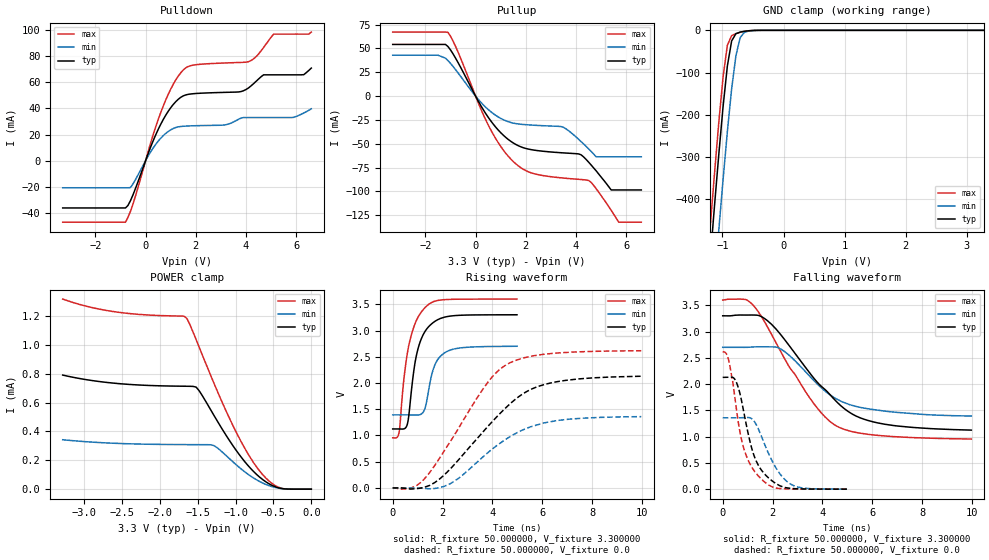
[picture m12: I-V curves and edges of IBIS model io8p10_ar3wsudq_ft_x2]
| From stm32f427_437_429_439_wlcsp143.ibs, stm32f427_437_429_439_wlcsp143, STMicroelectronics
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|   Model io8p10_ar3wsudq_ft_x2
[Model]  io8p10_ar3wsudq_ft_x2
Model_type I/O
Polarity   Non-Inverting
Enable   Active-Low
Vinl =   0.990000V
Vinh =   2.310000V
Vmeas =  1.650000V
Cref =   40.000000pF
Rref =   100.000000M
Vref =   0.0V
C_comp   7.528700pF   7.342900pF   7.752900pF
[Temperature Range]   25.000000   0.125000k   -40.000000
[Pullup Reference]   3.300000V   2.700000V   3.600000V
[Pulldown Reference]   0.0V   0.0V   0.0V
[POWER Clamp Reference]   3.300000V   2.700000V   3.600000V
[GND Clamp Reference]   0.0V   0.0V   0.0V
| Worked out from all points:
|   slope of the pulldown table from 0 to 0.495 V, typ, clamps not added: 20.9 ohm
|   slope of the pullup table from 0 to 0.495 V, typ, clamps not added: 22.6 ohm
|   GND clamp passes 1 mA (typ) near -0.57 V on its own axis
|   rising waveform, R_fixture 50.000000, V_fixture 3.300000: 20-80 % time 482ps typ, 432ps min, 512ps max; typ from 1.12 V to 3.3 V
|   rising waveform, R_fixture 50.000000, V_fixture 0.0: 20-80 % time 2.52ns typ, 2.27ns min, 2.13ns max; typ from 0 V to 2.13 V
|   falling waveform, R_fixture 50.000000, V_fixture 3.300000: 20-80 % time 2.35ns typ, 1.93ns min, 2.08ns max; typ from 3.3 V to 1.12 V
|   falling waveform, R_fixture 50.000000, V_fixture 0.0: 20-80 % time 718ps typ, 844ps min, 663ps max; typ from 2.13 V to 0 V
[Pulldown]
|Voltage   I(typ)   I(min)   I(max)
-3.3V     -36.18mA   -20.77mA   -47.07mA
-800mV    -36.18mA   -20.77mA   -47.07mA
-600mV    -30.5mA    -20.52mA   -38.69mA
700mV     31.4mA     19.11mA    41.71mA
1.2V      45.15mA    25.37mA    61.75mA
1.6V      50.35mA    26.5mA     71.06mA
3.1V      52.28mA    27.26mA    74.75mA
4.1V      55.71mA    33.01mA    75.8mA
4.7V      65.73mA    33.01mA    86.69mA
5.1V      65.73mA    33.01mA    96.9mA
6.3V      65.85mA    36.5mA     96.9mA
6.6V      70.91mA    39.71mA    98.45mA
[Pullup]
|Voltage   I(typ)   I(min)   I(max)
-3.3V     54.22mA    42.91mA    67.16mA
-1.1V     51.99mA    37.3mA     66.87mA
500mV     -22.07mA   -14mA      -30.03mA
1.5V      -49.1mA    -28.3mA    -68.56mA
2.2V      -56.05mA   -30.32mA   -80.35mA
3.5V      -59.53mA   -32.72mA   -85.92mA
4.2V      -61.52mA   -47.7mA    -87.46mA
4.5V      -69.21mA   -55.3mA    -88.43mA
4.8V      -78.3mA    -63.6mA    -97.02mA
5.4V      -98.4mA    -63.6mA    -119.8mA
5.7V      -98.4mA    -63.6mA    -132.2mA
6.6V      -98.4mA    -63.6mA    -132.2mA
[GND_clamp]
|Voltage   I(typ)   I(min)   I(max)
-3.3V     -4.652A    -4.81A     -4.601A
-1.2V     -540.3mA   -722.7mA   -464.2mA
-1.13V    -414.5mA   -596.2mA   -338mA
-1.06V    -293.4mA   -472.4mA   -217.6mA
-990mV    -180.4mA   -352.9mA   -109.9mA
-920mV    -84.42mA   -240mA     -35.36mA
-850mV    -25.15mA   -138.9mA   -12.53mA
-780mV    -7.942mA   -60.01mA   -7.772mA
-710mV    -4.199mA   -17.23mA   -4.763mA
-640mV    -2.296mA   -4.566mA   -2.439mA
-570mV    -1.048mA   -1.643mA   -953.6uA
3.28V     0A         0A         0A
[POWER_clamp]
|Voltage   I(typ)   I(min)   I(max)
-3.28V    790.5uA    342.5uA    1.317mA
-2.6V     734.3uA    318.1uA    1.23mA
-1.68V    713.4uA    308.8uA    1.199mA
-1.64V    713.1uA    308.7uA    1.182mA
-1.52V    707.2uA    308.5uA    1.037mA
-1.48V    682.1uA    308.4uA    984.7uA
-1.28V    507.2uA    300.7uA    728.4uA
-960mV    246.2uA    155.1uA    363.1uA
-720mV    101uA      64.07uA    152.4uA
-560mV    37.87uA    24.53uA    57.3uA
-440mV    10.21uA    7.381uA    14.65uA
0V        0A         0A         0A
[Ramp]
| variable   typ   min   max
dV/dt_r  1.26570/2.50561n   0.80886/2.25031n   1.56324/2.12207n
dV/dt_f  1.28142/2.33437n   0.77238/1.90340n   1.57424/2.07286n
R_load = 50.000000
[Rising Waveform]
R_fixture= 50.000000
V_fixture= 3.300000
V_fixture_min= 2.700000
V_fixture_max= 3.600000
|time   V(typ)   V(min)   V(max)
0s        1.124V     1.392V     954.2mV
260.3ps   1.124V     1.392V     1.069V
430.4ps   1.124V     1.392V     1.99V
570.6ps   1.19V      1.392V     2.517V
720.7ps   1.722V     1.391V     2.868V
940.9ps   2.503V     1.389V     3.182V
1.301ns   2.986V     1.528V     3.439V
1.672ns   3.168V     2.323V     3.555V
2.082ns   3.255V     2.575V     3.588V
4.985ns   3.3V       2.7V       3.599V
[Rising Waveform]
R_fixture= 50.000000
V_fixture= 0.0
V_fixture_min= 0.0
V_fixture_max= 0.0
|time   V(typ)   V(min)   V(max)
0s        324.9uV    179uV      1.453mV
780.8ps   -19.72mV   527.7uV    7.326mV
1.241ns   8.808mV    -7.85mV    157.8mV
1.682ns   101.2mV    -10.01mV   425.3mV
2.302ns   359.5mV    79.81mV    879.2mV
3.744ns   1.134V     643.5mV    1.967V
4.625ns   1.567V     954mV      2.366V
5.465ns   1.86V      1.153V     2.501V
6.366ns   2.004V     1.265V     2.561V
9.97ns    2.129V     1.359V     2.614V
[Falling Waveform]
R_fixture= 50.000000
V_fixture= 3.300000
V_fixture_min= 2.700000
V_fixture_max= 3.600000
|time   V(typ)   V(min)   V(max)
0s        3.3V       2.7V       3.599V
981ps     3.314V     2.7V       3.596V
1.301ns   3.314V     2.709V     3.458V
1.782ns   3.212V     2.709V     3.099V
2.482ns   2.847V     2.619V     2.483V
3.463ns   2.229V     2.164V     1.756V
4.565ns   1.666V     1.718V     1.203V
5.325ns   1.397V     1.577V     1.082V
6.226ns   1.26V      1.504V     1.024V
9.97ns    1.124V     1.392V     954.2mV
[Falling Waveform]
R_fixture= 50.000000
V_fixture= 0.0
V_fixture_min= 0.0
V_fixture_max= 0.0
|time   V(typ)   V(min)   V(max)
0s        2.129V     1.359V     2.614V
240.2ps   2.131V     1.359V     2.455V
550.6ps   2.032V     1.358V     1.521V
720.7ps   1.76V      1.359V     1.018V
890.9ps   1.357V     1.363V     709.2mV
1.171ns   767.1mV    1.339V     414.4mV
1.451ns   436.8mV    1.122V     240.9mV
2.122ns   110.2mV    415.6mV    23.51mV
2.653ns   19.85mV    118.5mV    4.842mV
4.985ns   324.9uV    179uV      1.453mV
